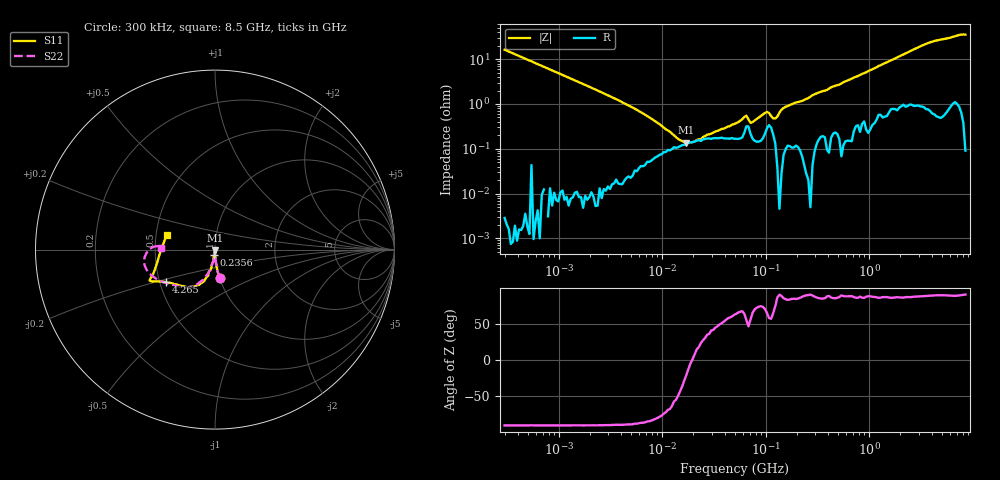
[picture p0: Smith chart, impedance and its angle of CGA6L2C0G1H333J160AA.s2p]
! S-parameter Generated by TDK Corporation
! Copyright(C) 2015 TDK Corporation.
! All Rights Reserved.
! TDK P/N: CGA6L2C0G1H333J160AA (Multilayer Ceramic Chip Capacitors)
! Property: C=33nF
! Size(LxWxT): 3.2x2.5x1.6mm, 0.126x0.098x0.063inches
! Model Type: s2p (Touchstone File Format Version 1.0)
! Frequency: DC=Yes Start=0.3MHz Stop=8500MHz 225points Log-sweep
! Note:
! Model Generated on Jun. 23, 2015
! Hash(MD5):
! Port Assignments:
!  1 ---| |--- 2
! Applicable Conditions:
!  Temperature = 25 degC
!  DC Bias Voltage = 0 V
!  Small Signal Operation
! Terms and conditions regarding TDK Simulation Models
! (1)This simulation model is being provided solely for informational purposes. Please refer to the specifications of the products in terms of detailed characteristics of such products.
! (2)In no event shall TDK Corporation of any of its subsidiaries be liable for any loss or damage arising, directly or indirectly,
!  From any information contained in this simulation model, including, but not limited to loss or damages arising from any inaccuracies, omissions or errors in connection with such information.
! (3)Any and all copyrights on this simulation model are owned by TDK Corporation.
!  Duplication or redistribution of this simulation model without prior written permission from TDK Corporation is prohibited.
! (4)This simulation model is subject to any modification or change without any prior notice.
! (5)Neither TDK Corporation nor any of its subsidiaries shall make any warranty, express or implied,
!  Including but not limited to the correctness, implied warranties of merchantability and fitness for a particular purpose with respect to this simulation models.
! (6)The use of this simulation model shall be deemed to have consented to the terms and conditions hereof.
# MHz S MA R 50
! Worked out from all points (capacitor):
!   224 points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, 300 kHz to 8.5 GHz, reference 50 ohm
!   read as one part in series: C = 32.6 nF near 314.1 kHz
!   lowest |Z| = 138 mohm at 17.14 MHz (marker M1)
!   series resonance near 19.48 MHz, so ESL is about 2 nH
!   S11 on the Smith chart (normalised r, x): 300 kHz: 1.00, -0.33; 235.6 MHz: 0.99, -0.06; 4.265 GHz: 0.54, -0.22; 8.5 GHz: 0.57, +0.10
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0.3  0.1614 -80.7  0.9868 9.2  0.9869 9.3  0.1614 -80.8
1.72111  0.02828 -88.4  0.9996 1.6  0.9995 1.6  0.02827 -88.3
9.430415  0.005132 -85.8  0.9992 0.1  0.9991 0.1  0.005452 -80.6
12.42578  0.004064 -83.2  0.999 -0.0  0.9988 -0.0  0.004695 -74.9
17.1428  0.003358 -80.2  0.9986 -0.2  0.9984 -0.2  0.004543 -68.8
29.76236  0.003256 -84.0  0.9981 -0.4  0.9978 -0.4  0.005855 -68.6
51.67171  0.004827 -98.4  0.9972 -0.8  0.9972 -0.8  0.008814 -79.1
62.1033  0.005393 -95.8  0.9963 -1.0  0.9961 -0.9  0.00976 -79.1
71.28712  0.008588 -96.6  0.996 -1.0  0.996 -1.0  0.01281 -83.9
98.34885  0.01128 -97.4  0.9953 -1.4  0.9952 -1.4  0.0145 -89.5
123.7646  0.01794 -96.2  0.9958 -1.6  0.9957 -1.6  0.01963 -95.9
142.0669  0.01952 -100.9  0.9971 -2.0  0.9969 -1.9  0.01918 -96.4
235.5662  0.03097 -101.7  0.9945 -3.2  0.9945 -3.2  0.03189 -99.9
283.1228  0.03771 -100.9  0.9942 -3.9  0.994 -3.8  0.03448 -100.7
514.6664  0.06812 -98.6  0.9922 -7.1  0.9919 -7.1  0.07023 -99.3
1551.304  0.1803 -109.0  0.9725 -20.9  0.9725 -20.8  0.1734 -111.6
2693.286  0.2537 -124.7  0.9475 -35.4  0.9476 -35.4  0.2548 -125.0
4265.177  0.3266 -146.3  0.9177 -54.6  0.9176 -54.6  0.3261 -144.8
5619.915  0.4003 -154.0  0.8898 -69.7  0.8898 -69.6  0.3977 -163.8
6754.475  0.3739 -157.8  0.8855 -81.3  0.8854 -81.3  0.381 -177.5
7404.957  0.3344 -166.0  0.8957 -88.3  0.8956 -88.3  0.3428 177.3
8500  0.2809 162.6  0.9053 -102.4  0.9054 -102.4  0.3013 178.7
